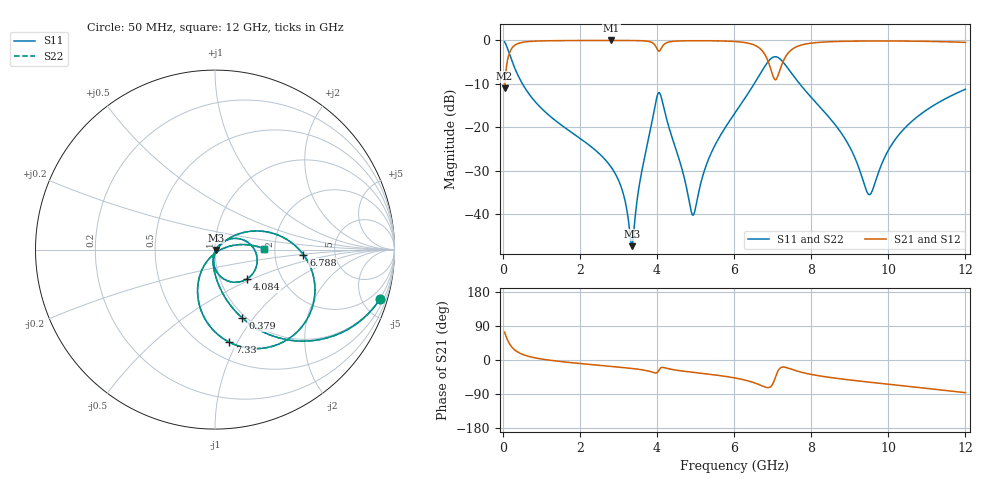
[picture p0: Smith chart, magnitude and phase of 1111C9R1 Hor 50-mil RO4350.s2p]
# GHz S MA R 50
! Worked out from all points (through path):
!   11951 points, 50 MHz to 12 GHz, reference 50 ohm
!   highest |S21| = -0.02 dB at 2.821 GHz (marker M1); lowest = -11.0 dB at 50 MHz (marker M2)
!   group delay of S21, straight-line fit = 21 ps
!   lowest |S11| = -47.4 dB at 3.35 GHz (marker M3), VSWR 1.01, Z = 50.4 - j0.205 ohm
!   |S11| at or under -10 dB: 511.2 MHz to 6.523 GHz (6.012 GHz wide, 171 % of centre); 7.701 GHz to end of sweep
!   |S22| runs from -47.4 to -0.4 dB; largest |S21 - S12| = 0
!   S11 on the Smith chart (normalised r, x): 50 MHz: 0.96, -6.71; 379 MHz: 0.96, -0.88; 4.084 GHz: 1.34, -0.47; 6.788 GHz: 2.93, -0.22; 7.33 GHz: 0.65, -0.93; 12 GHz: 1.75, +0.02
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0.05  0.9599 -16.6  0.2803 73.4  0.2803 73.4  0.9599 -16.6
0.178  0.6929 -47.3  0.7207 42.7  0.7207 42.7  0.6929 -47.3
0.379  0.4107 -68.2  0.9112 21.7  0.9112 21.7  0.4107 -68.2
2.042  0.07227 -98.6  0.9959 -9.6  0.9959 -9.6  0.07227 -98.6
2.821  0.03421 -103.6  0.9973 -17.0  0.9973 -17.0  0.03421 -103.6
3.12  0.01759 -100.8  0.9969 -19.9  0.9969 -19.9  0.01759 -100.8
3.35  0.004254 -28.6  0.9956 -22.4  0.9956 -22.4  0.004254 -28.6
3.59  0.02821 46.2  0.9906 -25.5  0.9906 -25.5  0.02821 46.2
4.034  0.2462 -17.8  0.7576 -29.7  0.7576 -29.7  0.2462 -17.8
4.084  0.2414 -42.9  0.7703 -22.2  0.7703 -22.2  0.2414 -42.9
4.286  0.1092 -88.9  0.9507 -22.7  0.9507 -22.7  0.1092 -88.9
4.932  0.009665 -31.3  0.9901 -32.5  0.9901 -32.5  0.009665 -31.3
5.362  0.04526 40.0  0.989 -37.6  0.989 -37.6  0.04526 40.0
6.025  0.146 34.7  0.9691 -47.4  0.9691 -47.4  0.146 34.7
6.788  0.4935 -3.3  0.7005 -70.7  0.7005 -70.7  0.4935 -3.3
7.069  0.648 -44.5  0.3518 -46.6  0.3518 -46.6  0.648 -44.5
7.33  0.5219 -81.2  0.6417 -19.3  0.6417 -19.3  0.5219 -81.2
8.017  0.2168 -116.0  0.9307 -38.3  0.9307 -38.3  0.2168 -116.0
8.913  0.06927 -123.9  0.9763 -51.6  0.9763 -51.6  0.06927 -123.9
9.49  0.01683 -62.6  0.9828 -58.3  0.9828 -58.3  0.01683 -62.6
10.009  0.05491 10.3  0.9833 -64.0  0.9833 -64.0  0.05491 10.3
12  0.2734 1.0  0.9485 -86.3  0.9485 -86.3  0.2734 1.0
